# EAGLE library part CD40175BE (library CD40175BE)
Texas Instruments CD40175BE Quad D Type Flip Flop IC, CMOS, 16-Pin PDIP Source: Datasheet
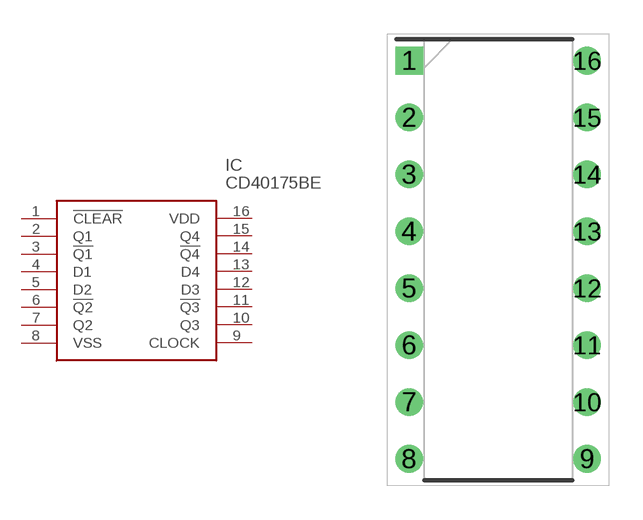
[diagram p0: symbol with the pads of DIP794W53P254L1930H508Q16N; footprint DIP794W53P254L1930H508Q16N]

Designator prefix IC

## CD40175BE (Description: Texas Instruments CD40175BE Quad D Type Flip Flop IC, CMOS, 16-Pin PDIP; Height: 5.08mm; Manufacturer_Name: Texas Instruments; Manufacturer_Part_Number: CD40175BE; Mouser_Part_Number: 595-CD40175BE; Mouser_Price-Stock: https://www.mouser.co.uk/ProductDetail/Texas-Instruments/CD40175BE?qs=0le1rQK8zxrp%252BJWBqTTnBw%3D%3D)  [DIP794W53P254L1930H508Q16N]
1  !CLEAR
2  Q1
3  !Q1
4  D1
5  D2
6  !Q2
7  Q2
8  VSS
9  CLOCK
10  Q3
11  !Q3
12  D3
13  D4
14  !Q4
15  Q4
16  VDD

## Footprint DIP794W53P254L1930H508Q16N (pad centres in mm)
N (R-PDIP-T)
drill 0.73 pad 1.13 square: 1 -3.97,8.89
drill 0.73 pad 1.13: 2 -3.97,6.35; 3 -3.97,3.81; 4 -3.97,1.27; 5 -3.97,-1.27; 6 -3.97,-3.81; 7 -3.97,-6.35; 8 -3.97,-8.89; 9 3.97,-8.89; 10 3.97,-6.35; 11 3.97,-3.81; 12 3.97,-1.27; 13 3.97,1.27; 14 3.97,3.81; 15 3.97,6.35; 16 3.97,8.89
